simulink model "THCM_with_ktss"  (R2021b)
settings: Solver=ode15s  StartTime=0.0  StopTime=100  RelTol=1e-3  EnableMultiTasking=on
StopFcn:
  | %
  | %  Get the necessary parameters from the model workspace:
  | %  ------------------------------------------------------
  | %
  | model_workspace = get_param(bdroot(gcs), 'ModelWorkspace');
  | T = getVariable(model_workspace, 'T');
  | b1 = getVariable(model_workspace, 'b1');
  | 
  | clear model_workspace
  | 
  | %
  | %  Recover the data needed to compute the transfer functions
  | %  TF_s(e^jw) = F_s(e^jw)/b_1*v_in1(e^jw) and
  | %  TF_us2(e^jw) = F_us2(e^jw)/b_1*v_in1(e^jw).
  | %  NOTE: The data are selected so that their lengths are the maximum
  | %  exact multiple of 2 permitted by the data for FFT (rather than DFT):
  | %  --------------------------------------------------------------------
  | %
  | data_len = numel(bond12.Time);
  | fft_len = 2^floor(log2(data_len));
  | 
  | %
  | %  Define Hann / Hamming window (see more at the following link:
  | %  https://en.wikipedia.org/wiki/List_of_window_functions#Cosine-sum_windows):
  | %  ---------------------------------------------------------------------------
  | %
  | N = fft_len - 1;
  | n = (0:N)';
  | wf = @(a0) (a0 - (1 - a0)*cos(2*pi*n/N));
  | %w = ones(fft_len, 1);
  | %w = wf(25/46);% Hamming
  | w = wf(0.5); % Hann
  | 
  | %
  | %  Extract the data from the timeseries object folowing a simulation run.
  | %  (Efforts, flows, and powers are in columns #1, #2, and #3 respectively.)
  | %  ------------------------------------------------------------------------
  | %
  | v_in1_data = bond01.Data(1:fft_len, 2);
  | F_s_data = bond12.Data(1:fft_len, 1);
  | F_us1_data = bond04.Data(1:fft_len, 1);
  | F_us2_data = bond19.Data(1:fft_len, 1);
  | 
  | TF_s_num_data = F_s_data;
  | TF_s_den_data = v_in1_data*b1;
  | 
  | TF_us1_num_data = F_us1_data;
  | TF_us1_den_data = v_in1_data*b1;
  | 
  | TF_us2_num_data = F_us2_data;
  | TF_us2_den_data = v_in1_data*b1;
  | 
  | clear F_s_data F_us1_data F_us2_data v_in1_data b1
  | 
  | %
  | %  Window the data prior to taking FFTs to reduce effects
  | %  of spectral leakage due to finite-duration sequences:
  | %  -----------------------------------------------------
  | %
  | TF_s_num_data_w = TF_s_num_data.*w;
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model workspace (MAT data in the model file):
  T = 0.001
  b = 1964
  b1 = 1964
  b2 = 1964
  g0 = 9.80665
  k = 220000
  k1 = 31500
  k2 = 31500
  k_t1 = 220000
  k_t2 = 220000
  m_s = 680
  m_s_s0 = -0.141970693354
  m_us1 = 40
  m_us2 = 40
undefined symbols (not defined in the file): Frequency, Junction, Limited, Parallel, Series
libraries: lib_simbus_extras x16, lib_connector x11, lib_generic_capacitance x5, lib_zero_junction x5, lib_one_junction x5, lib_generic_inertance x3, lib_effort_source x3, lib_generic_resistance x3, lib_time_derivative x2, lib_modulated_flow_source x1, lib_select_power_variable x1, simulink x1

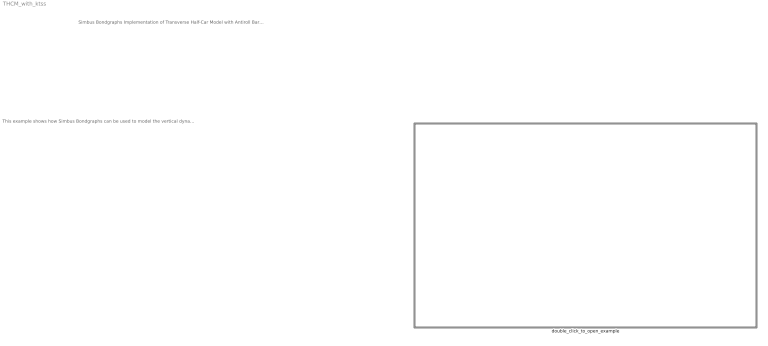
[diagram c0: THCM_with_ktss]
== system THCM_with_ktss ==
  note: This example shows how Simbus Bondgraphs can be used to model the vertical dynamics of a car that combines a damper with the traditional antiroll bar. This arrangement is used in the Koenigsegg Triplex Suspension System pioneered by Koenigsegg for high-performance supercars. Hector Medina and Natasha Carpenter show in their paper " Transverse Third-Damper to Improve Suspension Systems for In-Wheel Motor Driven Electric Vehicles " that the third damper offers better road-holding for electric vehicles that have in-wheel motors (which therefore have larger unsprung masses than their nonelectric counterparts). The other advantage of the third damper is that it is a passive device and does not require energy-consuming active control. The transfer functions specified in the paper are plotted following completion of a simulation run. The bond graph and parameters are taken from the paper. These parameters are stored in the model's workspace and can be changed to see the effect on the transfer functions. The bond numbering used in the paper is also replicated in this model. The companion model to this model should also be consulted to see how the additional damper augments the dynamics.
  note: Simbus Bondgraphs Implementation of Transverse Half-Car Model with Antiroll Bar and Transverse Damper v2
  double_click_to_open_example : Subsystem

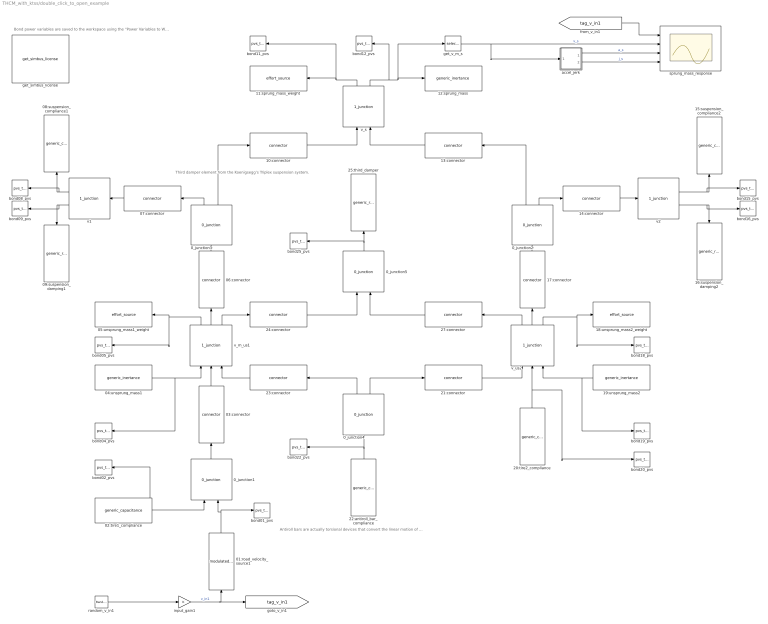
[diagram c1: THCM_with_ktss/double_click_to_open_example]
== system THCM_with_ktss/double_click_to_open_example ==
  note: Bond power variables are saved to the workspace using the "Power Variables to Workspace" blocks. The variablea are named "bondXX" where XX is the bond number (the bond number makes up the initial part of the name of each bond).
  note: Antiroll bars are actually torsional devices that convert the linear motion of one spring to rotational displacement and then to a linear displacement on the opposite spring. This arrangement can be described using two transformer (TF) junctions on either side of the 0-junction. Since the antiroll device is symmetrical, it is possible to replace the torsional compliance and represent the antiroll bar using a linear compliance C- element.
  note: Third damper element from the Koenigsegg’s Triplex suspension system.
  01:road_velocity_source1 : lib_modulated_flow_source/modulated_flow_source  simbus_vendor=SIMBUS  simbus_toolbox=SIMBUS_BONDGRAPHS  simbus_component=BLOCKS  simbus_class=bond.1_port.modulated_flow_source  msk_physical_domain=Generic  msk_connection_point=A  msk_power_direction=B => A  msk_icon_type=Default  msk_icon_source=Flow\nSource
  02:tire1_compliance : lib_generic_capacitance/generic_capacitance  simbus_vendor=SIMBUS  simbus_toolbox=SIMBUS_BONDGRAPHS  simbus_component=BLOCKS  simbus_class=bond.1_port.generic_capacitance  msk_physical_domain=Generic  msk_connection_point=A  msk_computed_pv=Effort  msk_lock_causality=off  msk_computation_method=Linear Relation  msk_capacitance=1/k_t1  msk_effort_table=[0 0; 1 1]  msk_effort_interp_method=Linear point-slope  msk_effort_extrap_method=Linear  msk_displacement_table=[0 0; 1 1]  msk_displacement_interp_method=Linear point-slope  msk_displacement_extrap_method=Linear  msk_index_search_method=Binary search  msk_index_search_using_previous=on  msk_effort_expr=u  msk_displacement_expr=u  msk_int_tol=auto  msk_time_derivative_type=Simple  msk_highest_freq_hz=10  msk_freq_break_factor=2  msk_roll_off_factor=3  msk_q0=(m_s/2+m_us1)*g0/k_t1  msk_f0=0  msk_icon_type=Default  msk_icon_source=Generic\nCapacitance
  03:connector : lib_connector/connector  simbus_vendor=SIMBUS  simbus_toolbox=SIMBUS_BONDGRAPHS  simbus_component=BLOCKS  simbus_class=bond.connector.connector  msk_physical_domain=Generic  msk_power_direction=B => A  msk_causal_stroke_location=A  msk_lock_causality=off  msk_icon_type=Default  msk_icon_source=Connector
  04:unsprung_mass1 : lib_generic_inertance/generic_inertance  simbus_vendor=SIMBUS  simbus_toolbox=SIMBUS_BONDGRAPHS  simbus_component=BLOCKS  simbus_class=bond.1_port.generic_inertance  msk_physical_domain=Generic  msk_connection_point=A  msk_computed_pv=Flow  msk_lock_causality=off  msk_computation_method=Linear Relation  msk_inertance=m_us1  msk_momentum_table=[0 0; 1 1]  msk_momentum_interp_method=Linear point-slope  msk_momentum_extrap_method=Linear  msk_flow_table=[0 0; 1 1]  msk_flow_interp_method=Linear point-slope  msk_flow_extrap_method=Linear  msk_index_search_method=Binary search  msk_index_search_using_previous=on  msk_momentum_expr=(u>0.25)*u^(0.5)+(u<=0.25)*u^(1/3)  msk_flow_expr=u*sin(u)  msk_int_tol=auto  msk_time_derivative_type=Frequency-Limited  msk_highest_freq_hz=10  msk_freq_break_factor=2  msk_roll_off_factor=3  msk_p0=0  msk_e0=3  msk_icon_type=Default  msk_icon_source=Generic\nInertance
  05:unsprung_mass1_weight : lib_effort_source/effort_source  simbus_vendor=SIMBUS  simbus_toolbox=SIMBUS_BONDGRAPHS  simbus_component=BLOCKS  simbus_class=bond.1_port.effort_source  msk_physical_domain=Generic  msk_connection_point=B  msk_power_direction=B => A  msk_effort_value=m_us1*g0  msk_icon_type=Default  msk_icon_source=Effort\nSource
  06:connector : lib_connector/connector  simbus_vendor=SIMBUS  simbus_toolbox=SIMBUS_BONDGRAPHS  simbus_component=BLOCKS  simbus_class=bond.connector.connector  msk_physical_domain=Generic  msk_power_direction=B => A  msk_causal_stroke_location=B  msk_lock_causality=off  msk_icon_type=Default  msk_icon_source=Connector
  07:connector : lib_connector/connector  simbus_vendor=SIMBUS  simbus_toolbox=SIMBUS_BONDGRAPHS  simbus_component=BLOCKS  simbus_class=bond.connector.connector  msk_physical_domain=Generic  msk_power_direction=B => A  msk_causal_stroke_location=B  msk_lock_causality=off  msk_icon_type=Default  msk_icon_source=Connector
  08:suspension_compliance1 : lib_generic_capacitance/generic_capacitance  simbus_vendor=SIMBUS  simbus_toolbox=SIMBUS_BONDGRAPHS  simbus_component=BLOCKS  simbus_class=bond.1_port.generic_capacitance  msk_physical_domain=Generic  msk_connection_point=B  msk_computed_pv=Effort  msk_lock_causality=off  msk_computation_method=Linear Relation  msk_capacitance=1/k1  msk_effort_table=[0 0; 1 1]  msk_effort_interp_method=Linear point-slope  msk_effort_extrap_method=Linear  msk_displacement_table=[0 0; 1 1]  msk_displacement_interp_method=Linear point-slope  msk_displacement_extrap_method=Linear  msk_index_search_method=Binary search  msk_index_search_using_previous=on  msk_effort_expr=u  msk_displacement_expr=u  msk_int_tol=auto  msk_time_derivative_type=Simple  msk_highest_freq_hz=10  msk_freq_break_factor=2  msk_roll_off_factor=3  msk_q0=(m_s*g0/2)/k1  msk_f0=0  msk_icon_type=Default  msk_icon_source=Generic\nCapacitance
  09:suspension_damping1 : lib_generic_resistance/generic_resistance  simbus_vendor=SIMBUS  simbus_toolbox=SIMBUS_BONDGRAPHS  simbus_component=BLOCKS  simbus_class=bond.1_port.generic_resistance  msk_physical_domain=Generic  msk_connection_point=B  msk_computed_pv=Effort  msk_lock_causality=off  msk_computation_method=Linear Relation  msk_resistance=b1  msk_effort_table=[0 0; 1 1]  msk_effort_interp_method=Linear point-slope  msk_effort_extrap_method=Linear  msk_flow_table=[0 0; 1 1]  msk_flow_interp_method=Linear point-slope  msk_flow_extrap_method=Linear  msk_index_search_method=Linear search  msk_index_search_using_previous=on  msk_effort_expr=u  msk_flow_expr=u*sin(u)  msk_icon_type=Default  msk_icon_source=Generic\nResistance
  0_junction1 : lib_zero_junction/0_junction  simbus_vendor=SIMBUS  simbus_toolbox=SIMBUS_BONDGRAPHS  simbus_component=BLOCKS  simbus_class=bond.3_port.0_junction  msk_physical_domain=Generic  msk_num_a_side_ports=2  msk_num_b_side_ports=1  msk_icon_type=Default  msk_icon_source=0-Junction\n(Parallel Junction)
  0_junction2 : lib_zero_junction/0_junction  simbus_vendor=SIMBUS  simbus_toolbox=SIMBUS_BONDGRAPHS  simbus_component=BLOCKS  simbus_class=bond.3_port.0_junction  msk_physical_domain=Generic  msk_num_a_side_ports=1  msk_num_b_side_ports=2  msk_icon_type=Default  msk_icon_source=0-Junction\n(Parallel Junction)
  0_junction3 : lib_zero_junction/0_junction  simbus_vendor=SIMBUS  simbus_toolbox=SIMBUS_BONDGRAPHS  simbus_component=BLOCKS  simbus_class=bond.3_port.0_junction  msk_physical_domain=Generic  msk_num_a_side_ports=1  msk_num_b_side_ports=2  msk_icon_type=Default  msk_icon_source=0-Junction\n(Parallel Junction)
  0_junction4 : lib_zero_junction/0_junction  simbus_vendor=SIMBUS  simbus_toolbox=SIMBUS_BONDGRAPHS  simbus_component=BLOCKS  simbus_class=bond.3_port.0_junction  msk_physical_domain=Generic  msk_num_a_side_ports=1  msk_num_b_side_ports=2  msk_icon_type=Default  msk_icon_source=0-Junction\n(Parallel Junction)
  0_junction5 : lib_zero_junction/0_junction  simbus_vendor=SIMBUS  simbus_toolbox=SIMBUS_BONDGRAPHS  simbus_component=BLOCKS  simbus_class=bond.3_port.0_junction  msk_physical_domain=Generic  msk_num_a_side_ports=2  msk_num_b_side_ports=1  msk_icon_type=Default  msk_icon_source=0-Junction\n(Parallel Junction)
  10:connector : lib_connector/connector  simbus_vendor=SIMBUS  simbus_toolbox=SIMBUS_BONDGRAPHS  simbus_component=BLOCKS  simbus_class=bond.connector.connector  msk_physical_domain=Generic  msk_power_direction=B => A  msk_causal_stroke_location=A  msk_lock_causality=off  msk_icon_type=Default  msk_icon_source=Connector
  11:sprung_mass_weight : lib_effort_source/effort_source  simbus_vendor=SIMBUS  simbus_toolbox=SIMBUS_BONDGRAPHS  simbus_component=BLOCKS  simbus_class=bond.1_port.effort_source  msk_physical_domain=Generic  msk_connection_point=B  msk_power_direction=B => A  msk_effort_value=m_s*g0  msk_icon_type=Default  msk_icon_source=Effort\nSource
  12:sprung_mass : lib_generic_inertance/generic_inertance  simbus_vendor=SIMBUS  simbus_toolbox=SIMBUS_BONDGRAPHS  simbus_component=BLOCKS  simbus_class=bond.1_port.generic_inertance  msk_physical_domain=Generic  msk_connection_point=B  msk_computed_pv=Flow  msk_lock_causality=off  msk_computation_method=Linear Relation  msk_inertance=m_s  msk_momentum_table=[0 0; 1 1]  msk_momentum_interp_method=Linear point-slope  msk_momentum_extrap_method=Linear  msk_flow_table=[0 0; 1 1]  msk_flow_interp_method=Linear point-slope  msk_flow_extrap_method=Linear  msk_index_search_method=Binary search  msk_index_search_using_previous=on  msk_momentum_expr=(u>0.25)*u^(0.5)+(u<=0.25)*u^(1/3)  msk_flow_expr=u*sin(u)  msk_int_tol=auto  msk_time_derivative_type=Frequency-Limited  msk_highest_freq_hz=10  msk_freq_break_factor=2  msk_roll_off_factor=3  msk_p0=0  msk_e0=3  msk_icon_type=Default  msk_icon_source=Generic\nInertance
  13:connector : lib_connector/connector  simbus_vendor=SIMBUS  simbus_toolbox=SIMBUS_BONDGRAPHS  simbus_component=BLOCKS  simbus_class=bond.connector.connector  msk_physical_domain=Generic  msk_power_direction=B => A  msk_causal_stroke_location=A  msk_lock_causality=off  msk_icon_type=Default  msk_icon_source=Connector
  14:connector : lib_connector/connector  simbus_vendor=SIMBUS  simbus_toolbox=SIMBUS_BONDGRAPHS  simbus_component=BLOCKS  simbus_class=bond.connector.connector  msk_physical_domain=Generic  msk_power_direction=B => A  msk_causal_stroke_location=B  msk_lock_causality=off  msk_icon_type=Default  msk_icon_source=Connector
  15:suspension_compliance2 : lib_generic_capacitance/generic_capacitance  simbus_vendor=SIMBUS  simbus_toolbox=SIMBUS_BONDGRAPHS  simbus_component=BLOCKS  simbus_class=bond.1_port.generic_capacitance  msk_physical_domain=Generic  msk_connection_point=B  msk_computed_pv=Effort  msk_lock_causality=off  msk_computation_method=Linear Relation  msk_capacitance=1/k2  msk_effort_table=[0 0; 1 1]  msk_effort_interp_method=Linear point-slope  msk_effort_extrap_method=Linear  msk_displacement_table=[0 0; 1 1]  msk_displacement_interp_method=Linear point-slope  msk_displacement_extrap_method=Linear  msk_index_search_method=Binary search  msk_index_search_using_previous=on  msk_effort_expr=u  msk_displacement_expr=u  msk_int_tol=auto  msk_time_derivative_type=Simple  msk_highest_freq_hz=10  msk_freq_break_factor=2  msk_roll_off_factor=3  msk_q0=(m_s*g0/2)/k2  msk_f0=0  msk_icon_type=Default  msk_icon_source=Generic\nCapacitance
  16:suspension_damping2 : lib_generic_resistance/generic_resistance  simbus_vendor=SIMBUS  simbus_toolbox=SIMBUS_BONDGRAPHS  simbus_component=BLOCKS  simbus_class=bond.1_port.generic_resistance  msk_physical_domain=Generic  msk_connection_point=B  msk_computed_pv=Effort  msk_lock_causality=off  msk_computation_method=Linear Relation  msk_resistance=b2  msk_effort_table=[0 0; 1 1]  msk_effort_interp_method=Linear point-slope  msk_effort_extrap_method=Linear  msk_flow_table=[0 0; 1 1]  msk_flow_interp_method=Linear point-slope  msk_flow_extrap_method=Linear  msk_index_search_method=Linear search  msk_index_search_using_previous=on  msk_effort_expr=u  msk_flow_expr=u*sin(u)  msk_icon_type=Default  msk_icon_source=Generic\nResistance
  17:connector : lib_connector/connector  simbus_vendor=SIMBUS  simbus_toolbox=SIMBUS_BONDGRAPHS  simbus_component=BLOCKS  simbus_class=bond.connector.connector  msk_physical_domain=Generic  msk_power_direction=B => A  msk_causal_stroke_location=B  msk_lock_causality=off  msk_icon_type=Default  msk_icon_source=Connector
  18:unsprung_mass2_weight : lib_effort_source/effort_source  simbus_vendor=SIMBUS  simbus_toolbox=SIMBUS_BONDGRAPHS  simbus_component=BLOCKS  simbus_class=bond.1_port.effort_source  msk_physical_domain=Generic  msk_connection_point=B  msk_power_direction=B => A  msk_effort_value=m_us2*g0  msk_icon_type=Default  msk_icon_source=Effort\nSource
  19:unsprung_mass2 : lib_generic_inertance/generic_inertance  simbus_vendor=SIMBUS  simbus_toolbox=SIMBUS_BONDGRAPHS  simbus_component=BLOCKS  simbus_class=bond.1_port.generic_inertance  msk_physical_domain=Generic  msk_connection_point=A  msk_computed_pv=Flow  msk_lock_causality=off  msk_computation_method=Linear Relation  msk_inertance=m_us2  msk_momentum_table=[0 0; 1 1]  msk_momentum_interp_method=Linear point-slope  msk_momentum_extrap_method=Linear  msk_flow_table=[0 0; 1 1]  msk_flow_interp_method=Linear point-slope  msk_flow_extrap_method=Linear  msk_index_search_method=Binary search  msk_index_search_using_previous=on  msk_momentum_expr=(u>0.25)*u^(0.5)+(u<=0.25)*u^(1/3)  msk_flow_expr=u*sin(u)  msk_int_tol=auto  msk_time_derivative_type=Frequency-Limited  msk_highest_freq_hz=10  msk_freq_break_factor=2  msk_roll_off_factor=3  msk_p0=0  msk_e0=3  msk_icon_type=Default  msk_icon_source=Generic\nInertance
  20:tire2_compliance : lib_generic_capacitance/generic_capacitance  simbus_vendor=SIMBUS  simbus_toolbox=SIMBUS_BONDGRAPHS  simbus_component=BLOCKS  simbus_class=bond.1_port.generic_capacitance  msk_physical_domain=Generic  msk_connection_point=A  msk_computed_pv=Effort  msk_lock_causality=off  msk_computation_method=Linear Relation  msk_capacitance=1/k_t2  msk_effort_table=[0 0; 1 1]  msk_effort_interp_method=Linear point-slope  msk_effort_extrap_method=Linear  msk_displacement_table=[0 0; 1 1]  msk_displacement_interp_method=Linear point-slope  msk_displacement_extrap_method=Linear  msk_index_search_method=Binary search  msk_index_search_using_previous=on  msk_effort_expr=u  msk_displacement_expr=u  msk_int_tol=auto  msk_time_derivative_type=Simple  msk_highest_freq_hz=10  msk_freq_break_factor=2  msk_roll_off_factor=3  msk_q0=(m_s/2+m_us2)*g0/k_t2  msk_f0=0  msk_icon_type=Default  msk_icon_source=Generic\nCapacitance
  21:connector : lib_connector/connector  simbus_vendor=SIMBUS  simbus_toolbox=SIMBUS_BONDGRAPHS  simbus_component=BLOCKS  simbus_class=bond.connector.connector  msk_physical_domain=Generic  msk_power_direction=B => A  msk_causal_stroke_location=A  msk_lock_causality=off  msk_icon_type=Default  msk_icon_source=Connector
  22:antiroll_bar_compliance : lib_generic_capacitance/generic_capacitance  simbus_vendor=SIMBUS  simbus_toolbox=SIMBUS_BONDGRAPHS  simbus_component=BLOCKS  simbus_class=bond.1_port.generic_capacitance  msk_physical_domain=Generic  msk_connection_point=A  msk_computed_pv=Effort  msk_lock_causality=off  msk_computation_method=Linear Relation  msk_capacitance=1/k  msk_effort_table=[0 0; 1 1]  msk_effort_interp_method=Linear point-slope  msk_effort_extrap_method=Linear  msk_displacement_table=[0 0; 1 1]  msk_displacement_interp_method=Linear point-slope  msk_displacement_extrap_method=Linear  msk_index_search_method=Binary search  msk_index_search_using_previous=on  msk_effort_expr=u  msk_displacement_expr=u  msk_int_tol=auto  msk_time_derivative_type=Simple  msk_highest_freq_hz=10  msk_freq_break_factor=2  msk_roll_off_factor=3  msk_q0=0  msk_f0=0  msk_icon_type=Default  msk_icon_source=Generic\nCapacitance
  23:connector : lib_connector/connector  simbus_vendor=SIMBUS  simbus_toolbox=SIMBUS_BONDGRAPHS  simbus_component=BLOCKS  simbus_class=bond.connector.connector  msk_physical_domain=Generic  msk_power_direction=B <= A  msk_causal_stroke_location=A  msk_lock_causality=off  msk_icon_type=Default  msk_icon_source=Connector
  24:connector : lib_connector/connector  simbus_vendor=SIMBUS  simbus_toolbox=SIMBUS_BONDGRAPHS  simbus_component=BLOCKS  simbus_class=bond.connector.connector  msk_physical_domain=Generic  msk_power_direction=B => A  msk_causal_stroke_location=B  msk_lock_causality=off  msk_icon_type=Default  msk_icon_source=Connector
  25:third_damper : lib_generic_resistance/generic_resistance  simbus_vendor=SIMBUS  simbus_toolbox=SIMBUS_BONDGRAPHS  simbus_component=BLOCKS  simbus_class=bond.1_port.generic_resistance  msk_physical_domain=Generic  msk_connection_point=B  msk_computed_pv=Effort  msk_lock_causality=off  msk_computation_method=Linear Relation  msk_resistance=b  msk_effort_table=[0 0; 1 1]  msk_effort_interp_method=Linear point-slope  msk_effort_extrap_method=Linear  msk_flow_table=[0 0; 1 1]  msk_flow_interp_method=Linear point-slope  msk_flow_extrap_method=Linear  msk_index_search_method=Linear search  msk_index_search_using_previous=on  msk_effort_expr=u  msk_flow_expr=u*sin(u)  msk_icon_type=Default  msk_icon_source=Generic\nResistance
  27:connector : lib_connector/connector  simbus_vendor=SIMBUS  simbus_toolbox=SIMBUS_BONDGRAPHS  simbus_component=BLOCKS  simbus_class=bond.connector.connector  msk_physical_domain=Generic  msk_power_direction=B <= A  msk_causal_stroke_location=B  msk_lock_causality=off  msk_icon_type=Default  msk_icon_source=Connector
  accel_jerk : Subsystem  mask(Compute Acceleration and Jerk){msk_highest_freq_hz=1000, msk_freq_break_factor=1, msk_roll_off_factor=1, msk_int_tol=auto}
      mask prompts: msk_highest_freq_hz "Highest Frequency in Signal (Hz):"; msk_freq_break_factor "Derivative Roll-Off Break Frequency (Multiple of Above):"; msk_roll_off_factor "Derivative Roll-Off Factor:"; msk_int_tol "Absolute Integration Tolerance:"
      mask help: Computes the acceleration and jerk as the output signals given the velocity as the input signal.
  bond01_pvs : lib_simbus_extras/pvs_to_workspace  simbus_vendor=SIMBUS  simbus_toolbox=SIMBUS_BONDGRAPHS  simbus_component=BLOCKS  simbus_class=measurement.pvs_to_workspace  msk_var_name=bond01  msk_max_datapoints=inf  msk_decimation=1  msk_save_format=Timeseries  msk_sample_time=T  msk_apply_antialiasing=on
  bond02_pvs : lib_simbus_extras/pvs_to_workspace  simbus_vendor=SIMBUS  simbus_toolbox=SIMBUS_BONDGRAPHS  simbus_component=BLOCKS  simbus_class=measurement.pvs_to_workspace  msk_var_name=bond02  msk_max_datapoints=inf  msk_decimation=1  msk_save_format=Timeseries  msk_sample_time=T  msk_apply_antialiasing=on
  bond04_pvs : lib_simbus_extras/pvs_to_workspace  simbus_vendor=SIMBUS  simbus_toolbox=SIMBUS_BONDGRAPHS  simbus_component=BLOCKS  simbus_class=measurement.pvs_to_workspace  msk_var_name=bond04  msk_max_datapoints=inf  msk_decimation=1  msk_save_format=Timeseries  msk_sample_time=T  msk_apply_antialiasing=on
  bond05_pvs : lib_simbus_extras/pvs_to_workspace  simbus_vendor=SIMBUS  simbus_toolbox=SIMBUS_BONDGRAPHS  simbus_component=BLOCKS  simbus_class=measurement.pvs_to_workspace  msk_var_name=bond05  msk_max_datapoints=inf  msk_decimation=1  msk_save_format=Timeseries  msk_sample_time=T  msk_apply_antialiasing=on
  bond08_pvs : lib_simbus_extras/pvs_to_workspace  simbus_vendor=SIMBUS  simbus_toolbox=SIMBUS_BONDGRAPHS  simbus_component=BLOCKS  simbus_class=measurement.pvs_to_workspace  msk_var_name=bond08  msk_max_datapoints=inf  msk_decimation=1  msk_save_format=Timeseries  msk_sample_time=T  msk_apply_antialiasing=on
  bond09_pvs : lib_simbus_extras/pvs_to_workspace  simbus_vendor=SIMBUS  simbus_toolbox=SIMBUS_BONDGRAPHS  simbus_component=BLOCKS  simbus_class=measurement.pvs_to_workspace  msk_var_name=bond09  msk_max_datapoints=inf  msk_decimation=1  msk_save_format=Timeseries  msk_sample_time=T  msk_apply_antialiasing=on
  bond11_pvs : lib_simbus_extras/pvs_to_workspace  simbus_vendor=SIMBUS  simbus_toolbox=SIMBUS_BONDGRAPHS  simbus_component=BLOCKS  simbus_class=measurement.pvs_to_workspace  msk_var_name=bond11  msk_max_datapoints=inf  msk_decimation=1  msk_save_format=Timeseries  msk_sample_time=T  msk_apply_antialiasing=on
  bond12_pvs : lib_simbus_extras/pvs_to_workspace  simbus_vendor=SIMBUS  simbus_toolbox=SIMBUS_BONDGRAPHS  simbus_component=BLOCKS  simbus_class=measurement.pvs_to_workspace  msk_var_name=bond12  msk_max_datapoints=inf  msk_decimation=1  msk_save_format=Timeseries  msk_sample_time=T  msk_apply_antialiasing=on
  bond15_pvs : lib_simbus_extras/pvs_to_workspace  simbus_vendor=SIMBUS  simbus_toolbox=SIMBUS_BONDGRAPHS  simbus_component=BLOCKS  simbus_class=measurement.pvs_to_workspace  msk_var_name=bond15  msk_max_datapoints=inf  msk_decimation=1  msk_save_format=Timeseries  msk_sample_time=T  msk_apply_antialiasing=on
  bond16_pvs : lib_simbus_extras/pvs_to_workspace  simbus_vendor=SIMBUS  simbus_toolbox=SIMBUS_BONDGRAPHS  simbus_component=BLOCKS  simbus_class=measurement.pvs_to_workspace  msk_var_name=bond16  msk_max_datapoints=inf  msk_decimation=1  msk_save_format=Timeseries  msk_sample_time=T  msk_apply_antialiasing=on
  bond18_pvs : lib_simbus_extras/pvs_to_workspace  simbus_vendor=SIMBUS  simbus_toolbox=SIMBUS_BONDGRAPHS  simbus_component=BLOCKS  simbus_class=measurement.pvs_to_workspace  msk_var_name=bond18  msk_max_datapoints=inf  msk_decimation=1  msk_save_format=Timeseries  msk_sample_time=T  msk_apply_antialiasing=on
  bond19_pvs : lib_simbus_extras/pvs_to_workspace  simbus_vendor=SIMBUS  simbus_toolbox=SIMBUS_BONDGRAPHS  simbus_component=BLOCKS  simbus_class=measurement.pvs_to_workspace  msk_var_name=bond19  msk_max_datapoints=inf  msk_decimation=1  msk_save_format=Timeseries  msk_sample_time=T  msk_apply_antialiasing=on
  bond20_pvs : lib_simbus_extras/pvs_to_workspace  simbus_vendor=SIMBUS  simbus_toolbox=SIMBUS_BONDGRAPHS  simbus_component=BLOCKS  simbus_class=measurement.pvs_to_workspace  msk_var_name=bond20  msk_max_datapoints=inf  msk_decimation=1  msk_save_format=Timeseries  msk_sample_time=T  msk_apply_antialiasing=on
  bond22_pvs : lib_simbus_extras/pvs_to_workspace  simbus_vendor=SIMBUS  simbus_toolbox=SIMBUS_BONDGRAPHS  simbus_component=BLOCKS  simbus_class=measurement.pvs_to_workspace  msk_var_name=bond22  msk_max_datapoints=inf  msk_decimation=1  msk_save_format=Timeseries  msk_sample_time=T  msk_apply_antialiasing=on
  bond25_pvs : lib_simbus_extras/pvs_to_workspace  simbus_vendor=SIMBUS  simbus_toolbox=SIMBUS_BONDGRAPHS  simbus_component=BLOCKS  simbus_class=measurement.pvs_to_workspace  msk_var_name=bond25  msk_max_datapoints=inf  msk_decimation=1  msk_save_format=Timeseries  msk_sample_time=T  msk_apply_antialiasing=on
  get_simbus_license : lib_simbus_extras/get_simbus_license  simbus_vendor=SIMBUS  simbus_toolbox=SIMBUS_CORE  simbus_component=BLOCKS  simbus_class=core.utils.get_simbus_license
  get_v_m_s : lib_select_power_variable/select_power_variable  simbus_vendor=SIMBUS  simbus_toolbox=SIMBUS_BONDGRAPHS  simbus_component=BLOCKS  simbus_class=measurement.select_power_variable  msk_pv_name=Flow  msk_bond_idx=1  msk_multibond_connected=logical(false)
  input_gain1 : Gain
  random_v_in1 : simulink/Sources/Band-Limited White Noise  Cov=[0.01]  Ts=10*T  seed=6781
  sprung_mass_response : Scope  NumInputPorts=4
  v1 : lib_one_junction/1_junction  simbus_vendor=SIMBUS  simbus_toolbox=SIMBUS_BONDGRAPHS  simbus_component=BLOCKS  simbus_class=bond.3_port.1_junction  msk_physical_domain=Generic  msk_num_a_side_ports=1  msk_num_b_side_ports=2  msk_icon_type=Default  msk_icon_source=1-Junction\n(Series Junction)
  v2 : lib_one_junction/1_junction  simbus_vendor=SIMBUS  simbus_toolbox=SIMBUS_BONDGRAPHS  simbus_component=BLOCKS  simbus_class=bond.3_port.1_junction  msk_physical_domain=Generic  msk_num_a_side_ports=1  msk_num_b_side_ports=2  msk_icon_type=Default  msk_icon_source=1-Junction\n(Series Junction)
  v_m_us1 : lib_one_junction/1_junction  simbus_vendor=SIMBUS  simbus_toolbox=SIMBUS_BONDGRAPHS  simbus_component=BLOCKS  simbus_class=bond.3_port.1_junction  msk_physical_domain=Generic  msk_num_a_side_ports=3  msk_num_b_side_ports=3  msk_icon_type=Default  msk_icon_source=1-Junction\n(Series Junction)
  v_s : lib_one_junction/1_junction  simbus_vendor=SIMBUS  simbus_toolbox=SIMBUS_BONDGRAPHS  simbus_component=BLOCKS  simbus_class=bond.3_port.1_junction  msk_physical_domain=Generic  msk_num_a_side_ports=2  msk_num_b_side_ports=2  msk_icon_type=Default  msk_icon_source=1-Junction\n(Series Junction)
  v_us2 : lib_one_junction/1_junction  simbus_vendor=SIMBUS  simbus_toolbox=SIMBUS_BONDGRAPHS  simbus_component=BLOCKS  simbus_class=bond.3_port.1_junction  msk_physical_domain=Generic  msk_num_a_side_ports=3  msk_num_b_side_ports=3  msk_icon_type=Default  msk_icon_source=1-Junction\n(Series Junction)
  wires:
  14:connector/1 -> v2/1
  0_junction2/2 -> 14:connector/1
  17:connector/1 -> 0_junction2/1
  0_junction2/1 -> 13:connector/1
  v_s/1 -> bond11_pvs/1, 11:sprung_mass_weight/1
  0_junction3/2 -> 10:connector/1
  06:connector/1 -> 0_junction3/1
  07:connector/1 -> v1/1
  04:unsprung_mass1/1 -> bond04_pvs/1, v_m_us1/1
  0_junction3/1 -> 07:connector/1
  0_junction1/1 -> 03:connector/1
  03:connector/1 -> v_m_us1/2
  01:road_velocity_source1/1 -> 0_junction1/2, bond01_pvs/1
  02:tire1_compliance/1 -> bond02_pvs/1, 0_junction1/1
  0_junction4/1 -> 23:connector/1
  0_junction4/2 -> 21:connector/1
  v_us2/2 -> 17:connector/1
  19:unsprung_mass2/1 -> bond19_pvs/1, v_us2/3
  v1/1 -> bond08_pvs/1, 08:suspension_compliance1/1
  v1/2 -> 09:suspension_damping1/1, bond09_pvs/1
  v2/1 -> bond15_pvs/1, 15:suspension_compliance2/1
  v2/2 -> bond16_pvs/1, 16:suspension_damping2/1
  [tag_v_in1] -> sprung_mass_response/1
  v_s/2 -> bond12_pvs/1, get_v_m_s/1, 12:sprung_mass/1
  get_v_m_s/1 -> accel_jerk/1(in_v), sprung_mass_response/2  "v_s"
  accel_jerk/1(out_a) -> sprung_mass_response/3  "a_s"
  v_m_us1/1 -> bond05_pvs/1, 05:unsprung_mass1_weight/1
  13:connector/1 -> v_s/2
  10:connector/1 -> v_s/1
  input_gain1/1 -> 01:road_velocity_source1/1, [tag_v_in1]  "v_in1"
  21:connector/1 -> v_us2/1
  20:tire2_compliance/1 -> bond20_pvs/1, v_us2/2
  v_us2/3 -> bond18_pvs/1, 18:unsprung_mass2_weight/1
  random_v_in1/1 -> input_gain1/1
  accel_jerk/2(out_j) -> sprung_mass_response/4  "j_s"
  22:antiroll_bar_compliance/1 -> 0_junction4/1, bond22_pvs/1
  23:connector/1 -> v_m_us1/3
  v_m_us1/2 -> 06:connector/1
  v_m_us1/3 -> 24:connector/1
  24:connector/1 -> 0_junction5/1
  27:connector/1 -> 0_junction5/2
  v_us2/1 -> 27:connector/1
  0_junction5/1 -> 25:third_damper/1, bond25_pvs/1

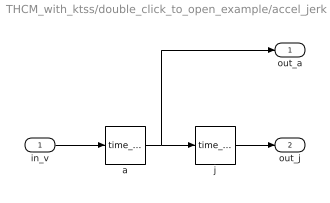
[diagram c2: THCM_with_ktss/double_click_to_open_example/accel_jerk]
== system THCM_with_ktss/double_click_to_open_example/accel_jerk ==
  in_v : Inport  PortDimensions=1
  a : lib_time_derivative/time_derivative  simbus_vendor=SIMBUS  simbus_toolbox=SIMBUS_CORE  simbus_component=BLOCKS  simbus_class=core.linear.time_derivative  msk_time_derivative_type=Frequency-Limited  msk_highest_freq_hz=msk_highest_freq_hz  msk_freq_break_factor=msk_freq_break_factor  msk_roll_off_factor=msk_roll_off_factor  msk_u0=0  msk_y0=0  msk_int_tol=auto
  j : lib_time_derivative/time_derivative  simbus_vendor=SIMBUS  simbus_toolbox=SIMBUS_CORE  simbus_component=BLOCKS  simbus_class=core.linear.time_derivative  msk_time_derivative_type=Frequency-Limited  msk_highest_freq_hz=msk_highest_freq_hz  msk_freq_break_factor=msk_freq_break_factor  msk_roll_off_factor=msk_roll_off_factor  msk_u0=0  msk_y0=0  msk_int_tol=auto
  out_a : Outport  PortDimensions=1
  out_j : Outport  Port=2  PortDimensions=1
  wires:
  a/1 -> out_a/1, j/1
  in_v/1 -> a/1
  j/1 -> out_j/1
